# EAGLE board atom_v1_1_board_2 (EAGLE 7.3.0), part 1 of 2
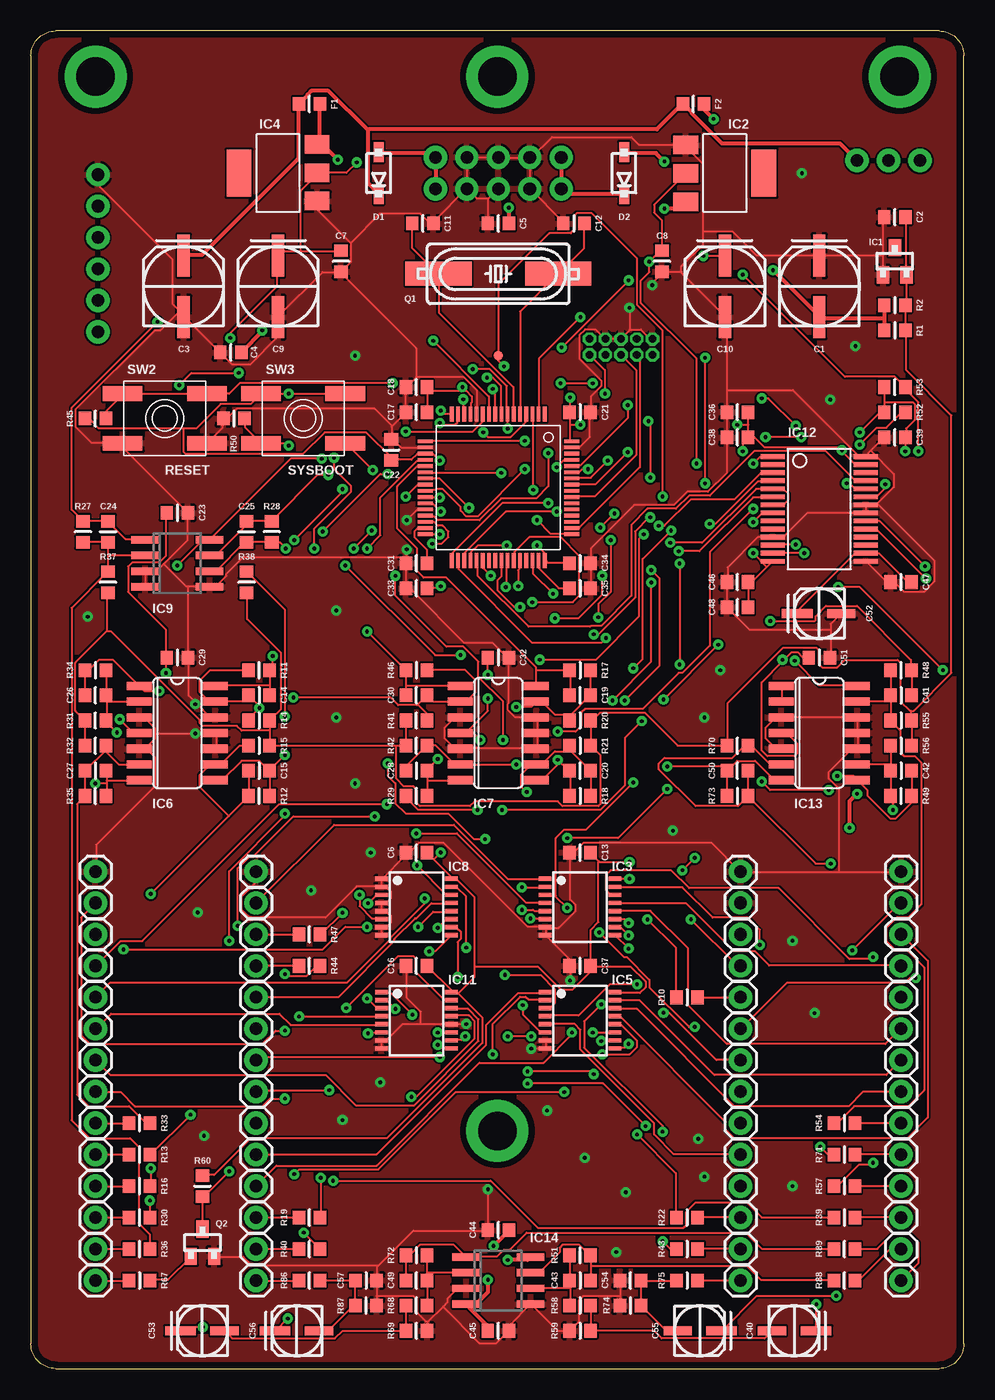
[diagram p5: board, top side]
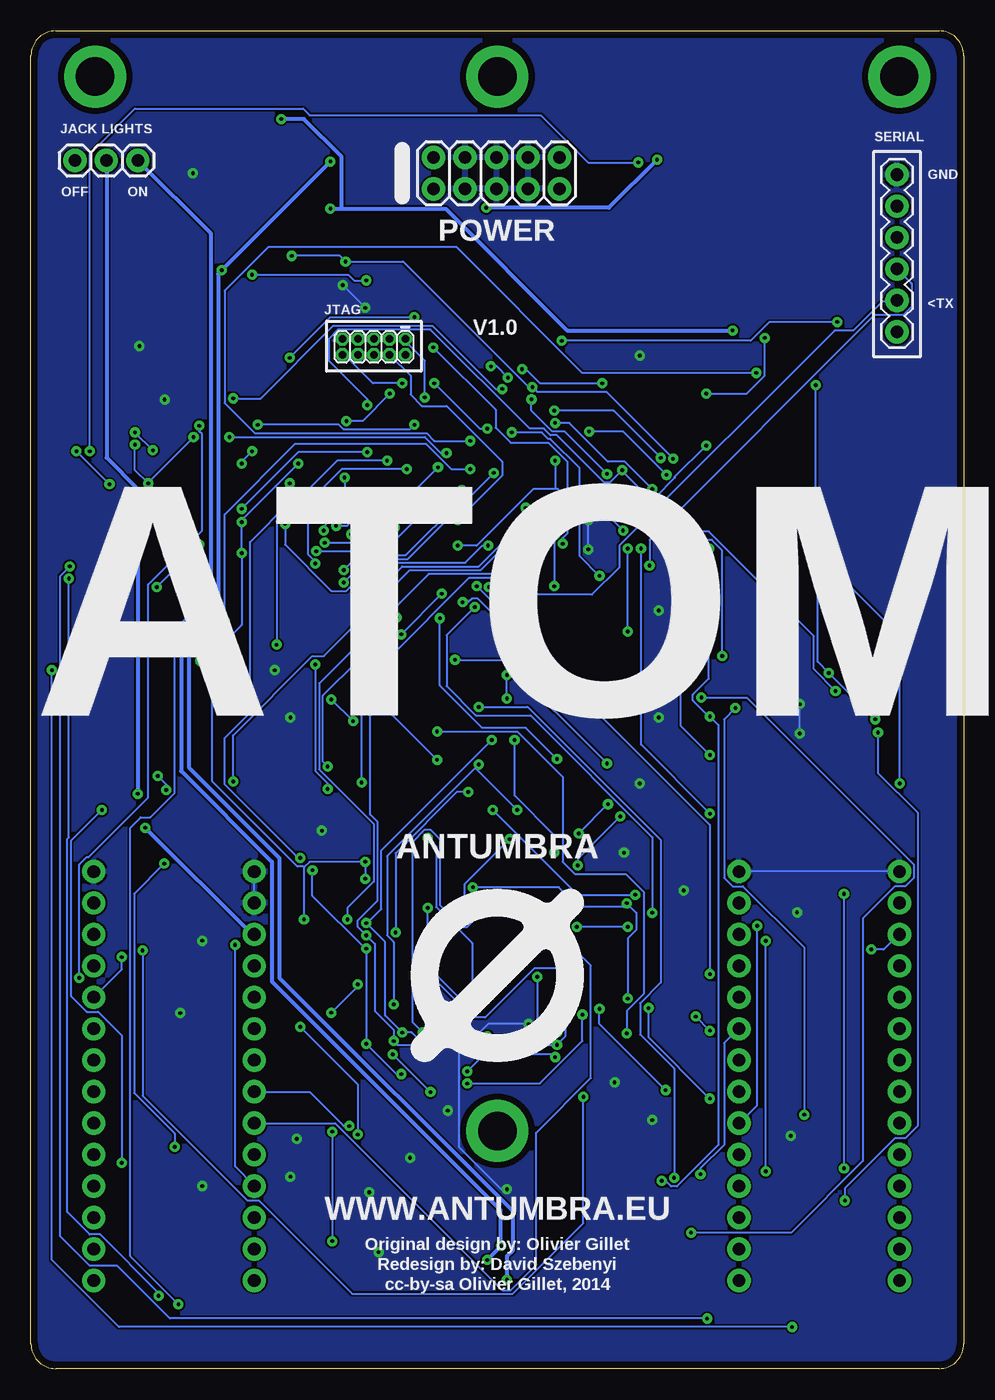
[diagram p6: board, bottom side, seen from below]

Size 75.3 x 108 mm. Coordinates in mm from the lower left corner, seen from the top.
Outline: 2,0 73.3,0 arc90 75.3,2 75.3,106 arc90 73.3,108 2,108 arc90 0,106 0,2 arc90 2,0
Copper layers (1*16): Top 0.035mm / dielectric 1.5mm / Bottom 0.035mm
Design rules "PCBCart-Standard": minimum track width 6mil, minimum drill 12mil, track to track 6mil, track to pad 6mil, pad to pad 6mil, via to via 6mil, smd to smd 6mil, copper to edge 20mil, drill to drill 8mil, minimum pad ring 8mil, minimum via ring 10mil, stop-mask expansion 3mil, vias tented up to drill 25mil, thermal gap 8mil
Net classes: 0 default: width 0.152 mm, drill 0.305 mm, clearance 0.152 mm; 1 wide: width 0.305 mm, drill 0.305 mm, clearance 0.305 mm

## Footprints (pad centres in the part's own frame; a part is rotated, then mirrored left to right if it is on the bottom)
PANASONIC_D = smd 3.4 x 1: + 2.478,0; - -2.478,0
RESISTOR_0603 = smd 1 x 1.1: 1 -0.85,0; 2 0.85,0
PANASONIC_B = smd 2.464 x 0.762: + 1.778,0 | smd 2.286 x 0.762: - -1.778,0
SOD123 = smd 1.6 x 0.8: + 1.7,0; - -1.7,0
PCB_SCREW = drill 3.1 pad 5: P$1 0,0
SOT23 = smd 1 x 1.4: 1 -0.95,-1.1; 2 0.95,-1.1; 3 0,1.1
SOT223 = smd 1.499 x 2.007: 1 -2.261,-3.15; 2 0.025,-3.15; 3 2.311,-3.15 | smd 3.81 x 2.007: 4 0,3.15
TSSOP16 = smd 0.35 x 1: 1 -1.95,-2.825; 2 -1.3,-2.825; 3 -0.65,-2.825; 4 0,-2.825; 5 0.65,-2.825; 6 1.3,-2.825; 7 1.95,-2.825; 8 2.6,-2.825; 9 2.6,2.825; 10 1.95,2.825; 11 1.3,2.825; 12 0.65,2.825; 13 0,2.825; 14 -0.65,2.825; 15 -1.3,2.825; 16 -1.95,2.825
SO14 = smd 0.66 x 2.032: 1 -3.81,-3.073; 2 -2.54,-3.073; 3 -1.27,-3.073; 4 0,-3.073; 5 1.27,-3.073; 6 2.54,-3.073; 7 3.81,-3.073; 8 3.81,3.073; 9 2.54,3.073; 10 1.27,3.073; 11 0,3.073; 12 -1.27,3.073; 13 -2.54,3.073; 14 -3.81,3.073
SO08 = smd 0.6 x 2.2: 1 -1.905,-2.6; 2 -0.635,-2.6; 3 0.635,-2.6; 4 1.905,-2.6; 5 1.905,2.6; 6 0.635,2.6; 7 -0.635,2.6; 8 -1.905,2.6
TQFP-10X10-64 = smd 1.2 x 0.3: 1 -5.936,3.75; 2 -5.936,3.25; 3 -5.936,2.75; 4 -5.936,2.25; 5 -5.936,1.75; 6 -5.936,1.25; 7 -5.936,0.75; 8 -5.936,0.25; 9 -5.936,-0.25; 10 -5.936,-0.75; 11 -5.936,-1.25; 12 -5.936,-1.75; 13 -5.936,-2.25; 14 -5.936,-2.75; 15 -5.936,-3.25; 16 -5.936,-3.75; 33 5.886,-3.75; 34 5.886,-3.25; 35 5.886,-2.75; 36 5.886,-2.25; 37 5.886,-1.75; 38 5.886,-1.25; 39 5.886,-0.75; 40 5.886,-0.25; 41 5.886,0.25; 42 5.886,0.75; 43 5.886,1.25; 44 5.886,1.75; 45 5.886,2.25; 46 5.886,2.75; 47 5.886,3.25; 48 5.886,3.75 | smd 0.3 x 1.2: 17 -3.75,-5.911; 18 -3.25,-5.911; 19 -2.75,-5.911; 20 -2.25,-5.911; 21 -1.75,-5.911; 22 -1.25,-5.911; 23 -0.75,-5.911; 24 -0.25,-5.911; 25 0.25,-5.911; 26 0.75,-5.911; 27 1.25,-5.911; 28 1.75,-5.911; 29 2.25,-5.911; 30 2.75,-5.911; 31 3.25,-5.911; 32 3.75,-5.911; 49 3.75,5.936; 50 3.25,5.936; 51 2.75,5.936; 52 2.25,5.936; 53 1.75,5.936; 54 1.25,5.936; 55 0.75,5.936; 56 0.25,5.936; 57 -0.25,5.936; 58 -0.75,5.936; 59 -1.25,5.936; 60 -1.75,5.936; 61 -2.25,5.936; 62 -2.75,5.936; 63 -3.25,5.936; 64 -3.75,5.936
SSOP28 = smd 0.381 x 1.905: 1 -4.55,-3.752; 2 -3.9,-3.752; 3 -3.25,-3.752; 4 -2.6,-3.752; 5 -1.95,-3.752; 6 -1.3,-3.752; 7 -0.65,-3.752; 8 0,-3.752; 9 0.65,-3.752; 10 1.3,-3.752; 11 1.95,-3.752; 12 2.6,-3.752; 13 3.25,-3.752; 14 3.9,-3.752; 15 3.9,3.752; 16 3.25,3.752; 17 2.6,3.752; 18 1.95,3.752; 19 1.3,3.752; 20 0.65,3.752; 21 0,3.752; 22 -0.65,3.752; 23 -1.3,3.752; 24 -1.95,3.752; 25 -2.6,3.752; 26 -3.25,3.752; 27 -3.9,3.752; 28 -4.55,3.752
2X5-1.27 = drill 0.61 pad 1.067 octagon: 1 -1.27,3.81; 2 0,3.81; 3 -1.27,2.54; 4 0,2.54; 5 -1.27,1.27; 6 0,1.27; 7 -1.27,0; 8 0,0; 9 -1.27,-1.27; 10 0,-1.27
1X06 = drill 1.016 pad 1.88: 1 0,0; 2 2.54,0; 3 5.08,0; 4 7.62,0; 5 10.16,0; 6 12.7,0
1X01 = drill 1.016 pad 1.88: 1 0,0
1X03 = drill 1.016 pad 1.88: 1 -2.54,0; 2 0,0; 3 2.54,0
POWER_10 = drill 1.016 pad 1.88: 1 -5.08,-1.27; 2 -5.08,1.27; 3 -2.54,-1.27; 4 -2.54,1.27; 5 0,-1.27; 6 0,1.27; 7 2.54,-1.27; 8 2.54,1.27; 9 5.08,-1.27; 10 5.08,1.27
HC49UP = smd 5.334 x 1.93: 1 -4.826,0; 2 4.826,0
EVQ-Q2 = smd 3.2 x 1.2: A -3.4,-2; A' 3.4,-2; B -3.4,2; B' 3.4,2
PAD.03X.03 = smd 0.762 x 0.762: P$1 0,0

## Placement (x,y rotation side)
C1  22u  [PANASONIC_D]  63.63,87.38 90 top
C2  100n  [RESISTOR_0603]  69.72,92.96 180 top
C3  22u  [PANASONIC_D]  12.32,87.38 90 top
C4  100n  [RESISTOR_0603]  16.13,82.04 180 top
C5  100n  [RESISTOR_0603]  37.72,92.46 180 top
C6  100n  [RESISTOR_0603]  31.12,41.66 180 top
C7  100n  [RESISTOR_0603]  25.02,89.41 270 top
C8  100n  [RESISTOR_0603]  50.93,89.41 270 top
C9  22u  [PANASONIC_D]  19.94,87.38 90 top
C10  22u  [PANASONIC_D]  56.01,87.38 90 top
C11  18p  [RESISTOR_0603]  31.62,92.46 180 top
C12  18p  [RESISTOR_0603]  43.82,92.46 0 top
C13  100n  [RESISTOR_0603]  44.32,41.66 180 top
C14  3.3n  [RESISTOR_0603]  18.42,54.36 0 top
C15  3.3n  [RESISTOR_0603]  18.42,48.26 0 top
C16  100n  [RESISTOR_0603]  31.12,32.51 180 top
C17  1u  [RESISTOR_0603]  31.12,77.22 180 top
C18  100n  [RESISTOR_0603]  31.12,79.25 180 top
C19  3.3n  [RESISTOR_0603]  44.32,54.36 180 top
C20  3.3n  [RESISTOR_0603]  44.32,48.26 180 top
C21  100n  [RESISTOR_0603]  44.32,77.22 0 top
C22  100n  [RESISTOR_0603]  29.08,74.17 90 top
C23  100n  [RESISTOR_0603]  11.81,69.09 0 top
C24  3.3n  [RESISTOR_0603]  6.22,67.56 90 top
C25  3.3n  [RESISTOR_0603]  17.4,67.56 90 top
C26  3.3n  [RESISTOR_0603]  5.21,54.36 180 top
C27  3.3n  [RESISTOR_0603]  5.21,48.26 0 top
C28  3.3n  [RESISTOR_0603]  31.12,48.26 0 top
C29  100n  [RESISTOR_0603]  11.81,57.4 0 top
C30  3.3n  [RESISTOR_0603]  31.12,54.36 180 top
C31  2.2u  [RESISTOR_0603]  31.12,65.02 180 top
C32  100n  [RESISTOR_0603]  37.72,57.4 0 top
C33  100n  [RESISTOR_0603]  31.12,62.99 180 top
C34  100n  [RESISTOR_0603]  44.32,65.02 0 top
C35  2.2u  [RESISTOR_0603]  44.32,62.99 0 top
C36  1u  [RESISTOR_0603]  57.02,77.22 180 top
C37  100n  [RESISTOR_0603]  44.32,32.51 180 top
C38  100n  [RESISTOR_0603]  57.02,75.18 180 top
C39  100n  [RESISTOR_0603]  69.72,75.18 180 top
C40  10u  [PANASONIC_B]  61.6,3.05 0 top
C41  3.3n  [RESISTOR_0603]  70.23,54.36 0 top
C42  3.3n  [RESISTOR_0603]  70.23,48.26 0 top
C43  18p  [RESISTOR_0603]  44.32,7.11 0 top
C44  100n  [RESISTOR_0603]  37.72,11.18 180 top
C45  100n  [RESISTOR_0603]  37.72,3.05 180 top
C46  100n  [RESISTOR_0603]  57.02,63.5 180 top
C47  100n  [RESISTOR_0603]  70.23,63.5 180 top
C48  1u  [RESISTOR_0603]  57.02,61.47 180 top
C49  18p  [RESISTOR_0603]  31.12,7.11 180 top
C50  3.3n  [RESISTOR_0603]  57.02,48.26 180 top
C51  100n  [RESISTOR_0603]  63.63,57.4 0 top
C52  10u  [PANASONIC_B]  63.63,60.96 180 top
C53  10u  [PANASONIC_B]  13.84,3.05 180 top
C54  220p  [RESISTOR_0603]  48.39,7.11 180 top
C55  10u  [PANASONIC_B]  53.98,3.05 0 top
C56  10u  [PANASONIC_B]  21.46,3.05 180 top
C57  220p  [RESISTOR_0603]  27.05,7.11 0 top
D1  1N5819HW  [SOD123]  28.07,96.52 90 top
D2  1N5819HW  [SOD123]  47.88,96.52 90 top
F1  FERRITE-BEAD  [RESISTOR_0603]  22.48,102.11 180 top
F2  FERRITE-BEAD  [RESISTOR_0603]  53.47,102.11 180 top
H1  PCB_SCREW  [PCB_SCREW]  5.22,104.31 0 top
H2  PCB_SCREW  [PCB_SCREW]  70.12,104.31 0 top
H3  PCB_SCREW  [PCB_SCREW]  37.65,104.31 0 top
H4  PCB_SCREW  [PCB_SCREW]  37.65,19.19 0 top
IC1  LM4040B10  [SOT23]  69.72,89.41 0 top
IC2  LM1117-3.3  [SOT223]  56.01,96.52 270 top
IC3  4051PW  [TSSOP16]  44.32,37.59 270 top
IC4  LM1117-3.3  [SOT223]  19.94,96.52 90 top
IC5  4051PW  [TSSOP16]  44.32,28.45 270 top
IC6  MCP6004  [SO14]  11.81,51.31 270 top
IC7  MCP6004  [SO14]  37.72,51.31 270 top
IC8  4051PW  [TSSOP16]  31.12,37.59 270 top
IC9  MCP6002  [SO08]  11.81,65.02 270 top
IC10  STM32F405RGT6  [TQFP-10X10-64]  37.72,71.12 270 top
IC11  4051PW  [TSSOP16]  31.12,28.45 270 top
IC12  WM8731  [SSOP28]  63.63,69.09 270 top
IC13  MCP6004  [SO14]  63.63,51.31 270 top
IC14  LME49720  [SO08]  37.72,7.11 270 top
JP1  M05X2MINIJTAG  [2X5-1.27]  48.9,81.85 270 bottom
JP2  [1X06]  5.4,96.39 270 bottom
JP3  [1X01]  5.21,40.13 0 top
JP4  [1X01]  18.16,40.13 0 top
JP5  [1X01]  57.28,7.11 0 top
JP6  [1X01]  57.28,40.13 0 top
JP7  [1X01]  18.16,7.11 0 top
JP8  [1X01]  70.23,40.13 0 top
JP9  [1X03]  69.22,97.54 0 bottom
JP10  [1X01]  70.23,9.65 0 top
JP11  [1X01]  70.23,7.11 0 top
JP25  [1X01]  5.21,9.65 0 top
JP26  [1X01]  70.23,12.19 0 top
JP27  [1X01]  5.21,12.19 0 top
JP28  [1X01]  5.21,17.27 0 top
JP29  [1X01]  5.21,14.73 0 top
JP30  [1X01]  5.21,19.81 0 top
JP31  [1X01]  18.16,9.65 0 top
JP32  [1X01]  18.16,12.19 0 top
JP33  [1X01]  57.28,12.19 0 top
JP34  [1X01]  57.28,9.65 0 top
JP35  [1X01]  70.23,19.81 0 top
JP36  [1X01]  70.23,14.73 0 top
JP37  [1X01]  70.23,17.27 0 top
JP65  [1X01]  70.23,37.59 0 top
JP66  [1X01]  5.21,24.89 0 top
JP67  [1X01]  5.21,22.35 0 top
JP68  [1X01]  57.28,22.35 0 top
JP69  [1X01]  5.21,27.43 0 top
JP70  [1X01]  18.16,22.35 0 top
JP71  [1X01]  5.21,37.59 0 top
JP72  [1X01]  18.16,29.97 0 top
JP73  [1X01]  18.16,19.81 0 top
JP74  [1X01]  57.28,19.81 0 top
JP75  [1X01]  5.21,35.05 0 top
JP76  [1X01]  70.23,35.05 0 top
JP77  [1X01]  70.23,22.35 0 top
JP78  [1X01]  70.23,24.89 0 top
JP79  [1X01]  18.16,27.43 0 top
JP80  [1X01]  18.16,17.27 0 top
JP81  [1X01]  57.28,17.27 0 top
JP82  [1X01]  18.16,24.89 0 top
JP83  [1X01]  57.28,24.89 0 top
JP84  [1X01]  70.23,32.51 0 top
JP85  [1X01]  70.23,29.97 0 top
JP86  [1X01]  57.28,14.73 0 top
JP87  [1X01]  70.23,27.43 0 top
JP88  [1X01]  18.16,37.59 0 top
JP89  [1X01]  18.16,14.73 0 top
JP90  [1X01]  5.21,29.97 0 top
JP91  [1X01]  5.21,32.51 0 top
JP93  [1X01]  5.21,7.11 0 top
JP94  [1X01]  57.28,27.43 0 top
JP95  [1X01]  57.28,29.97 0 top
JP100  [1X01]  18.16,35.05 0 top
JP101  [1X01]  18.16,32.51 0 top
JP102  [1X01]  57.28,32.51 0 top
JP103  [1X01]  57.28,37.59 0 top
JP107  [1X01]  57.28,35.05 0 top
P1  POWER_SIMPLE10  [POWER_10]  37.72,96.52 0 bottom
Q1  8MHz  [HC49UP]  37.72,88.39 0 top
Q2  MMBT3904  [SOT23]  13.84,10.16 0 top
R1  1.0k  [RESISTOR_0603]  69.72,83.82 0 top
R2  1.0k  [RESISTOR_0603]  69.72,85.85 0 top
R10  33  [RESISTOR_0603]  52.96,29.97 0 top
R11  20k  [RESISTOR_0603]  18.42,56.39 180 top
R12  20k  [RESISTOR_0603]  18.42,46.23 180 top
R13  100k  [RESISTOR_0603]  8.76,17.27 180 top
R14  120k  [RESISTOR_0603]  18.42,52.32 0 top
R15  120k  [RESISTOR_0603]  18.42,50.29 0 top
R16  100k  [RESISTOR_0603]  8.76,14.73 180 top
R17  20k  [RESISTOR_0603]  44.32,56.39 0 top
R18  20k  [RESISTOR_0603]  44.32,46.23 0 top
R19  100k  [RESISTOR_0603]  22.48,12.19 180 top
R20  120k  [RESISTOR_0603]  44.32,52.32 0 top
R21  120k  [RESISTOR_0603]  44.32,50.29 0 top
R22  100k  [RESISTOR_0603]  52.96,12.19 0 top
R27  47k  [RESISTOR_0603]  4.19,67.56 270 top
R28  20k  [RESISTOR_0603]  19.43,67.56 270 top
R29  20k  [RESISTOR_0603]  31.12,46.23 180 top
R30  100k  [RESISTOR_0603]  8.76,12.19 180 top
R31  200k  [RESISTOR_0603]  5.21,52.32 180 top
R32  120k  [RESISTOR_0603]  5.21,50.29 180 top
R33  100k  [RESISTOR_0603]  8.76,19.81 180 top
R34  33k  [RESISTOR_0603]  5.21,56.39 0 top
R35  20k  [RESISTOR_0603]  5.21,46.23 180 top
R36  100k  [RESISTOR_0603]  8.76,9.65 180 top
R37  180k  [RESISTOR_0603]  6.22,63.5 270 top
R38  120k  [RESISTOR_0603]  17.4,63.5 270 top
R39  100k  [RESISTOR_0603]  65.66,12.19 0 top
R40  100k  [RESISTOR_0603]  22.48,9.65 180 top
R41  120k  [RESISTOR_0603]  31.12,52.32 180 top
R42  120k  [RESISTOR_0603]  31.12,50.29 180 top
R43  100k  [RESISTOR_0603]  52.96,9.65 0 top
R44  2.2k  [RESISTOR_0603]  22.48,32.51 180 top
R45  10k  [RESISTOR_0603]  5.21,76.71 180 top
R46  20k  [RESISTOR_0603]  31.12,56.39 0 top
R47  2.2k  [RESISTOR_0603]  22.48,35.05 180 top
R48  20k  [RESISTOR_0603]  70.23,56.39 180 top
R49  20k  [RESISTOR_0603]  70.23,46.23 180 top
R50  10k  [RESISTOR_0603]  16.38,76.71 0 top
R51  47k  [RESISTOR_0603]  44.32,9.14 180 top
R52  2.2k  [RESISTOR_0603]  69.72,77.22 180 top
R53  2.2k  [RESISTOR_0603]  69.72,79.25 180 top
R54  100k  [RESISTOR_0603]  65.66,19.81 0 top
R55  120k  [RESISTOR_0603]  70.23,52.32 0 top
R56  120k  [RESISTOR_0603]  70.23,50.29 0 top
R57  100k  [RESISTOR_0603]  65.66,14.73 0 top
R58  6.8k  [RESISTOR_0603]  44.32,5.08 0 top
R59  47k  [RESISTOR_0603]  44.32,3.05 0 top
R60  10k  [RESISTOR_0603]  13.84,14.73 90 top
R67  100k  [RESISTOR_0603]  8.76,7.11 0 top
R68  6.8k  [RESISTOR_0603]  31.12,5.08 180 top
R69  47k  [RESISTOR_0603]  31.12,3.05 180 top
R70  120k  [RESISTOR_0603]  57.02,50.29 180 top
R71  100k  [RESISTOR_0603]  65.66,17.27 0 top
R72  47k  [RESISTOR_0603]  31.12,9.14 0 top
R73  20k  [RESISTOR_0603]  57.02,46.23 0 top
R74  6.8k  [RESISTOR_0603]  48.39,5.08 0 top
R75  36k  [RESISTOR_0603]  52.96,7.11 0 top
R86  36k  [RESISTOR_0603]  22.48,7.11 180 top
R87  6.8k  [RESISTOR_0603]  27.05,5.08 180 top
R88  1.0k  [RESISTOR_0603]  65.66,7.11 180 top
R89  1.0k  [RESISTOR_0603]  65.66,9.65 180 top
SW2  [EVQ-Q2]  10.8,76.71 0 top
SW3  [EVQ-Q2]  21.97,76.71 0 top
TP1  ADC_TEST  [PAD.03X.03]  37.72,81.79 0 top
U$1  [LOGO_14]  37.65,31.75 0 bottom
